PROGRAM Temp
VAR	
	H_LID				:ARRAY[1..10] OF Temp_controller;
	H_CHAMBER			:ARRAY[1..10] OF Temp_controller;
	H_PEN_VALVE			:Temp_controller;
	H_GATE_VALVE		:Temp_controller;
	H_IGS				:ARRAY[1..10] OF Temp_controller;
	H_TAPE				:ARRAY[1..10] OF Temp_controller;
	H_FORELINE			:ARRAY[1..20] OF Temp_controller;
	H_STAGE				:ARRAY[1..10] OF Temp_controller;	
END_VAR

//E01 PEN_VALVE PID		
	IF 	GV.AI.APC_Temp-GV.AO.APC_Temp_SV<3	
	THEN 
		H_PEN_VALVE.PID_Feedforward:=GV_H.PEN_VALVE_HEATER_PID.Feedforward;
	ELSE
		H_PEN_VALVE.PID_Feedforward:=0;
	END_IF	
	H_PEN_VALVE(
		ENABLE:= GV.AI.APC_Temp<110, 
		AUTO_TUNE:= GV.PEN_VALVE_HEATER_AUTO_TUNE_EN, 
		AUTO_TUNE_OUTPUT:=GV.PEN_VALVE_HEATER_AUTO_TUNE_OUTPUT,
		TEMP_SV:= GV.AO.APC_Temp_SV, 
		TEMP_ACTUAL:= GV.AI.APC_Temp, 
		TEMP_RATE:=5,
		PID_P:= GV_H.PEN_VALVE_HEATER_PID.P, 
		PID_I:= GV_H.PEN_VALVE_HEATER_PID.I, 
		PID_D:= GV_H.PEN_VALVE_HEATER_PID.D, 
		PID_Dp:= GV_H.PEN_VALVE_HEATER_PID.DP,
		PID_Output_Limit:= GV_H.PEN_VALVE_HEATER_PID.Output_Limit,
		SSR_ON=> GV.PEN_VALVE_HEATER_SSR_ON
	);		
	IF H_PEN_VALVE.PID_AUTO_TUNE_DONE
		THEN
		GV_H.PEN_VALVE_HEATER_PID.P:=H_PEN_VALVE.PID_AUTO_TUNE_P;
		GV_H.PEN_VALVE_HEATER_PID.I:=H_PEN_VALVE.PID_AUTO_TUNE_I;
		GV_H.PEN_VALVE_HEATER_PID.D:=H_PEN_VALVE.PID_AUTO_TUNE_D;
		GV.PEN_VALVE_HEATER_AUTO_TUNE_EN:=FALSE;
	END_IF
	
//E02 LID1 PID
	H_LID[1](
	ENABLE:= GV.AI.Lid_Temp<100, 
	AUTO_TUNE:= GV.LID_HEATER_AUTO_TUNE_EN[1], 
	AUTO_TUNE_OUTPUT:=GV.LID_HEATER_AUTO_TUNE_OUTPUT[1],
	TEMP_SV:= GV.AO.LID_Temp_SV, 
	TEMP_ACTUAL:= GV.AI.Lid_Temp, 
	TEMP_RATE:=5,
	PID_P:= GV_H.LID_HEATER_PID[1].P, 
	PID_I:= GV_H.LID_HEATER_PID[1].I, 
	PID_D:= GV_H.LID_HEATER_PID[1].D, 
	PID_Dp:= GV_H.LID_HEATER_PID[1].DP, 
	PID_Feedforward:= GV_H.LID_HEATER_PID[1].Feedforward,
	PID_Output_Limit:= GV_H.LID_HEATER_PID[1].Output_Limit,
	SSR_ON=> GV.LID_HEATER_SSR_ON[1],
	SSR_ON=> GV.LID_HEATER_SSR_ON[2],
	SSR_ON=> GV.LID_HEATER_SSR_ON[3],
	SSR_ON=> GV.LID_HEATER_SSR_ON[4]
	);	
	IF H_LID[1].PID_AUTO_TUNE_DONE
		THEN
		GV_H.LID_HEATER_PID[1].P:=H_LID[1].PID_AUTO_TUNE_P;
		GV_H.LID_HEATER_PID[1].I:=H_LID[1].PID_AUTO_TUNE_I;
		GV_H.LID_HEATER_PID[1].D:=H_LID[1].PID_AUTO_TUNE_D;
		GV.LID_HEATER_AUTO_TUNE_EN[1]:=FALSE;
	END_IF
//E06 CHAMBER1 PID
	H_CHAMBER[1](
	ENABLE:= GV.AI.CHAMBER_Temp1<100, 
	AUTO_TUNE:= GV.CHAMBER_HEATER_AUTO_TUNE_EN[1], 
	AUTO_TUNE_OUTPUT:=GV.CHAMBER_HEATER_AUTO_TUNE_OUTPUT[1],
	TEMP_SV:= GV.AO.Chamber_Temp1_SV, 
	TEMP_ACTUAL:= GV.AI.CHAMBER_Temp1, 
	TEMP_RATE:=5,
	PID_P:= GV_H.CHAMBER_HEATER_PID[1].P, 
	PID_I:= GV_H.CHAMBER_HEATER_PID[1].I, 
	PID_D:= GV_H.CHAMBER_HEATER_PID[1].D, 
	PID_Dp:= GV_H.CHAMBER_HEATER_PID[1].DP, 
	PID_Feedforward:= GV_H.CHAMBER_HEATER_PID[1].Feedforward,
	PID_Output_Limit:= GV_H.CHAMBER_HEATER_PID[1].Output_Limit,
	SSR_ON=> GV.CHAMBER_HEATER_SSR_ON[1]
	);	
	IF H_CHAMBER[1].PID_AUTO_TUNE_DONE
		THEN
		GV_H.CHAMBER_HEATER_PID[1].P:=H_CHAMBER[1].PID_AUTO_TUNE_P;
		GV_H.CHAMBER_HEATER_PID[1].I:=H_CHAMBER[1].PID_AUTO_TUNE_I;
		GV_H.CHAMBER_HEATER_PID[1].D:=H_CHAMBER[1].PID_AUTO_TUNE_D;
		GV.CHAMBER_HEATER_AUTO_TUNE_EN[1]:=FALSE;
	END_IF
//E07 CHAMBER2 PID	
	H_CHAMBER[2](
	ENABLE:= GV.AI.CHAMBER_Temp2<100, 
	AUTO_TUNE:= GV.CHAMBER_HEATER_AUTO_TUNE_EN[2], 
	AUTO_TUNE_OUTPUT:=GV.CHAMBER_HEATER_AUTO_TUNE_OUTPUT[2],
	TEMP_SV:= GV.AO.Chamber_Temp2_SV, 
	TEMP_ACTUAL:= GV.AI.CHAMBER_Temp2, 
	TEMP_RATE:=5,
	PID_P:= GV_H.CHAMBER_HEATER_PID[2].P, 
	PID_I:= GV_H.CHAMBER_HEATER_PID[2].I, 
	PID_D:= GV_H.CHAMBER_HEATER_PID[2].D, 
	PID_Dp:= GV_H.CHAMBER_HEATER_PID[2].DP, 
	PID_Feedforward:= GV_H.CHAMBER_HEATER_PID[2].Feedforward,
	PID_Output_Limit:= GV_H.CHAMBER_HEATER_PID[2].Output_Limit,
	SSR_ON=> GV.CHAMBER_HEATER_SSR_ON[2]
	);	
	IF H_CHAMBER[2].PID_AUTO_TUNE_DONE
		THEN
		GV_H.CHAMBER_HEATER_PID[2].P:=H_CHAMBER[2].PID_AUTO_TUNE_P;
		GV_H.CHAMBER_HEATER_PID[2].I:=H_CHAMBER[2].PID_AUTO_TUNE_I;
		GV_H.CHAMBER_HEATER_PID[2].D:=H_CHAMBER[2].PID_AUTO_TUNE_D;
		GV.CHAMBER_HEATER_AUTO_TUNE_EN[2]:=FALSE;
	END_IF
(*
	//E08 CHAMBER3 PID		
	H_CHAMBER[3](
	ENABLE:= GV.AI.CHAMBER_Temp3<100, 
	AUTO_TUNE:= GV.CHAMBER_HEATER_AUTO_TUNE_EN[3], 
	AUTO_TUNE_OUTPUT:=GV.CHAMBER_HEATER_AUTO_TUNE_OUTPUT[3],
	TEMP_SV:= GV.AO.Chamber_Temp3_SV, 
	TEMP_ACTUAL:= GV.AI.Chamber_Temp3, 
	PID_P:= GV_H.CHAMBER_HEATER_PID[3].P, 
	PID_I:= GV_H.CHAMBER_HEATER_PID[3].I, 
	PID_D:= GV_H.CHAMBER_HEATER_PID[3].D, 
	PID_Dp:= GV_H.CHAMBER_HEATER_PID[3].DP,
	PID_Feedforward:= GV_H.CHAMBER_HEATER_PID[3].Feedforward,
	PID_Output_Limit:= GV_H.CHAMBER_HEATER_PID[3].Output_Limit,
	SSR_ON=> GV.CHAMBER_HEATER_SSR_ON[4]
	);	
	IF H_CHAMBER[3].PID_AUTO_TUNE_DONE
		THEN
		GV_H.CHAMBER_HEATER_PID[3].P:=H_CHAMBER[3].PID_AUTO_TUNE_P;
		GV_H.CHAMBER_HEATER_PID[3].I:=H_CHAMBER[3].PID_AUTO_TUNE_I;
		GV_H.CHAMBER_HEATER_PID[3].D:=H_CHAMBER[3].PID_AUTO_TUNE_D;
		GV.CHAMBER_HEATER_AUTO_TUNE_EN[3]:=FALSE;
	END_IF

	//E18 GATE VALVE PID
		IF 	ABS(GV.AI.GATE_VALVE_Temp-GV.AO.Gate_Valve_Temp_SV)<5	
		THEN 
			H_GATE_VALVE.PID_Feedforward:=GV_H.GATE_VALVE_HEATER_PID.Feedforward;
		ELSE
			H_GATE_VALVE.PID_Feedforward:=0;
		END_IF
		H_GATE_VALVE(
		ENABLE:= GV.AI.GATE_VALVE_Temp<100, 
		AUTO_TUNE:= GV.GATE_VALVE_HEATER_AUTO_TUNE_EN, 
		AUTO_TUNE_OUTPUT:=GV.GATE_VALVE_HEATER_AUTO_TUNE_OUTPUT,
		TEMP_SV:= GV.AO.Gate_Valve_Temp_SV, 
		TEMP_ACTUAL:= GV.AI.GATE_VALVE_Temp, 
		PID_P:= GV_H.GATE_VALVE_HEATER_PID.P, 
		PID_I:= GV_H.GATE_VALVE_HEATER_PID.I, 
		PID_D:= GV_H.GATE_VALVE_HEATER_PID.D, 
		PID_Dp:= GV_H.GATE_VALVE_HEATER_PID.DP, 
		PID_Output_Limit:= GV_H.GATE_VALVE_HEATER_PID.Output_Limit,
		SSR_ON=> GV.GATE_VALVE_SSR_ON
		);		
		IF H_GATE_VALVE.PID_AUTO_TUNE_DONE
			THEN
			GV_H.GATE_VALVE_HEATER_PID.P:=H_GATE_VALVE.PID_AUTO_TUNE_P;
			GV_H.GATE_VALVE_HEATER_PID.I:=H_GATE_VALVE.PID_AUTO_TUNE_I;
			GV_H.GATE_VALVE_HEATER_PID.D:=H_GATE_VALVE.PID_AUTO_TUNE_D;
			GV.GATE_VALVE_HEATER_AUTO_TUNE_EN:=FALSE;
		END_IF	
		
	//E31	TAPE1 PID		
		H_TAPE[1](
		ENABLE:= GV.AI.TAPE_Temp1<120, 
		AUTO_TUNE:= GV.TAPE_HEATER_AUTO_TUNE_EN[1],
		AUTO_TUNE_OUTPUT:=GV.TAPE_HEATER_AUTO_TUNE_OUTPUT[1], 
		TEMP_SV:= GV.AO.Tape_Temp1_SV, 
		TEMP_ACTUAL:= GV.AI.TAPE_Temp1, 
		PID_P:= GV_H.TAPE_HEATER_PID[1].P, 
		PID_I:= GV_H.TAPE_HEATER_PID[1].I, 
		PID_D:= GV_H.TAPE_HEATER_PID[1].D, 
		PID_Dp:= GV_H.TAPE_HEATER_PID[1].DP, 
		PID_Feedforward:= ,
		PID_Output_Limit:= GV_H.TAPE_HEATER_PID[1].Output_Limit,
		SSR_ON=> GV.TAPE_HEATER_SSR_ON[1]
		);	
		IF H_TAPE[1].PID_AUTO_TUNE_DONE
			THEN
			GV_H.TAPE_HEATER_PID[1].P:=H_TAPE[1].PID_AUTO_TUNE_P;
			GV_H.TAPE_HEATER_PID[1].I:=H_TAPE[1].PID_AUTO_TUNE_I;
			GV_H.TAPE_HEATER_PID[1].D:=H_TAPE[1].PID_AUTO_TUNE_D;
			GV.TAPE_HEATER_AUTO_TUNE_EN[1]:=FALSE;
		END_IF
	//E32	TAPE2 PID		
		H_TAPE[2](
		ENABLE:= GV.AI.TAPE_Temp2<120, 
		AUTO_TUNE:= GV.TAPE_HEATER_AUTO_TUNE_EN[2], 
		AUTO_TUNE_OUTPUT:=GV.TAPE_HEATER_AUTO_TUNE_OUTPUT[2], 
		TEMP_SV:= GV.AO.Tape_Temp2_SV, 
		TEMP_ACTUAL:= GV.AI.TAPE_Temp2, 
		PID_P:= GV_H.TAPE_HEATER_PID[2].P, 
		PID_I:= GV_H.TAPE_HEATER_PID[2].I, 
		PID_D:= GV_H.TAPE_HEATER_PID[2].D, 
		PID_Dp:= GV_H.TAPE_HEATER_PID[2].DP, 
		PID_Feedforward:= ,
		PID_Output_Limit:= GV_H.TAPE_HEATER_PID[2].Output_Limit,
		SSR_ON=> GV.TAPE_HEATER_SSR_ON[2]
		);	
		IF H_TAPE[2].PID_AUTO_TUNE_DONE
			THEN
			GV_H.TAPE_HEATER_PID[2].P:=H_TAPE[2].PID_AUTO_TUNE_P;
			GV_H.TAPE_HEATER_PID[2].I:=H_TAPE[2].PID_AUTO_TUNE_I;
			GV_H.TAPE_HEATER_PID[2].D:=H_TAPE[2].PID_AUTO_TUNE_D;
			GV.TAPE_HEATER_AUTO_TUNE_EN[2]:=FALSE;
		END_IF
	//E35	IGS1 PID		
		H_IGS[1](
		ENABLE:= GV.AI.IGS_Temp1<50, 
		AUTO_TUNE:= GV.IGS_HEATER_AUTO_TUNE_EN[1], 
		AUTO_TUNE_OUTPUT:=GV.IGS_HEATER_AUTO_TUNE_OUTPUT[1], 
		TEMP_SV:= GV.AO.IGS_Temp1_SV, 
		TEMP_ACTUAL:= GV.AI.IGS_Temp1, 
		PID_P:= GV_H.IGS_HEATER_PID[1].P, 
		PID_I:= GV_H.IGS_HEATER_PID[1].I, 
		PID_D:= GV_H.IGS_HEATER_PID[1].D, 
		PID_Dp:= GV_H.IGS_HEATER_PID[1].DP, 
		PID_Feedforward:= GV_H.IGS_HEATER_PID[1].Feedforward,
		PID_Output_Limit:= GV_H.IGS_HEATER_PID[1].Output_Limit,
		SSR_ON=> GV.IGS_HEATER_SSR_ON[1]
		);	
		IF H_IGS[1].PID_AUTO_TUNE_DONE
			THEN
			GV_H.IGS_HEATER_PID[1].P:=H_IGS[1].PID_AUTO_TUNE_P;
			GV_H.IGS_HEATER_PID[1].I:=H_IGS[1].PID_AUTO_TUNE_I;
			GV_H.IGS_HEATER_PID[1].D:=H_IGS[1].PID_AUTO_TUNE_D;
			GV.IGS_HEATER_AUTO_TUNE_EN[1]:=FALSE;
		END_IF
	//E36	IGS2 PID	
		IF 	GV.AI.IGS_Temp2>GV.AO.IGS_Temp2_SV+3 THEN 
			H_IGS[2].PID_Feedforward:=0;
			ELSE
				H_IGS[2].PID_Feedforward:=GV_H.IGS_HEATER_PID[2].Feedforward;
		
		END_IF
		H_IGS[2](
		ENABLE:= GV.AI.IGS_Temp2<50, 
		AUTO_TUNE:= GV.IGS_HEATER_AUTO_TUNE_EN[2], 
		AUTO_TUNE_OUTPUT:=GV.IGS_HEATER_AUTO_TUNE_OUTPUT[2],
		TEMP_SV:= GV.AO.IGS_Temp2_SV, 
		TEMP_ACTUAL:= GV.AI.IGS_Temp2, 
		TEMP_RATE:=10,
		PID_P:= GV_H.IGS_HEATER_PID[2].P, 
		PID_I:= GV_H.IGS_HEATER_PID[2].I, 
		PID_D:= GV_H.IGS_HEATER_PID[2].D, 
		PID_Dp:= GV_H.IGS_HEATER_PID[2].DP, 
		PID_Feedforward:= ,
		PID_Output_Limit:= GV_H.IGS_HEATER_PID[2].Output_Limit,
		SSR_ON=> GV.IGS_HEATER_SSR_ON[2]
		);	
		IF H_IGS[2].PID_AUTO_TUNE_DONE
			THEN
			GV_H.IGS_HEATER_PID[2].P:=H_IGS[2].PID_AUTO_TUNE_P;
			GV_H.IGS_HEATER_PID[2].I:=H_IGS[2].PID_AUTO_TUNE_I;
			GV_H.IGS_HEATER_PID[2].D:=H_IGS[2].PID_AUTO_TUNE_D;
			GV.IGS_HEATER_AUTO_TUNE_EN[2]:=FALSE;
		END_IF
*)	
//FORELINE1 PID	SSR7	AV105	
	H_FORELINE[1](
	ENABLE:= GV.AI.AV105_Temp<120, 
	AUTO_TUNE:= GV.FORELINE_HEATER_AUTO_TUNE_EN[1], 
	AUTO_TUNE_OUTPUT:=GV.FORELINE_HEATER_AUTO_TUNE_OUTPUT[1],
	TEMP_SV:= GV.AO.AV105_Temp_SV, 
	TEMP_ACTUAL:= GV.AI.AV105_Temp, 
	TEMP_RATE:=10,
	PID_P:= GV_H.FORELINE_HEATER_PID[1].P, 
	PID_I:= GV_H.FORELINE_HEATER_PID[1].I, 
	PID_D:= GV_H.FORELINE_HEATER_PID[1].D, 
	PID_Dp:= GV_H.FORELINE_HEATER_PID[1].DP, 
	PID_Feedforward:= GV_H.FORELINE_HEATER_PID[1].Feedforward,
	PID_Output_Limit:= GV_H.FORELINE_HEATER_PID[1].Output_Limit,
	SSR_ON=> GV.FORELINE_HEATER_SSR_ON[1]);
	
	IF H_FORELINE[1].PID_AUTO_TUNE_DONE
		THEN
		GV_H.FORELINE_HEATER_PID[1].P:=H_FORELINE[1].PID_AUTO_TUNE_P;
		GV_H.FORELINE_HEATER_PID[1].I:=H_FORELINE[1].PID_AUTO_TUNE_I;
		GV_H.FORELINE_HEATER_PID[1].D:=H_FORELINE[1].PID_AUTO_TUNE_D;
		GV.FORELINE_HEATER_AUTO_TUNE_EN[1]:=FALSE;
	END_IF
//FORELINE2 PID		SSR8	AV104
	H_FORELINE[2](
	ENABLE:= GV.AI.AV104_Temp<120, 
	AUTO_TUNE:= GV.FORELINE_HEATER_AUTO_TUNE_EN[2], 
	AUTO_TUNE_OUTPUT:=GV.FORELINE_HEATER_AUTO_TUNE_OUTPUT[2],
	TEMP_SV:= GV.AO.AV104_Temp_SV, 
	TEMP_ACTUAL:= GV.AI.AV104_Temp,
	TEMP_RATE:=10, 
	PID_P:= GV_H.FORELINE_HEATER_PID[2].P, 
	PID_I:= GV_H.FORELINE_HEATER_PID[2].I, 
	PID_D:= GV_H.FORELINE_HEATER_PID[2].D, 
	PID_Dp:= GV_H.FORELINE_HEATER_PID[2].DP, 
	PID_Feedforward:= GV_H.FORELINE_HEATER_PID[2].Feedforward,
	PID_Output_Limit:= GV_H.FORELINE_HEATER_PID[2].Output_Limit,
	SSR_ON=> GV.FORELINE_HEATER_SSR_ON[2]);
	
	IF H_FORELINE[2].PID_AUTO_TUNE_DONE
		THEN
		GV_H.FORELINE_HEATER_PID[2].P:=H_FORELINE[2].PID_AUTO_TUNE_P;
		GV_H.FORELINE_HEATER_PID[2].I:=H_FORELINE[2].PID_AUTO_TUNE_I;
		GV_H.FORELINE_HEATER_PID[2].D:=H_FORELINE[2].PID_AUTO_TUNE_D;
		GV.FORELINE_HEATER_AUTO_TUNE_EN[2]:=FALSE;
	END_IF
//FORELINE3 PID		SSR9	AV102
IF GV.AI.AV102_Temp<GV.AO.AV102_Temp_SV+1
	THEN 
	GV_H.FORELINE_HEATER_PID[3].Feedforward:=8.5;
	ELSE
	GV_H.FORELINE_HEATER_PID[3].Feedforward:=0;
END_IF
	H_FORELINE[3](
	ENABLE:= GV.AI.AV102_Temp<120, 
	AUTO_TUNE:= GV.FORELINE_HEATER_AUTO_TUNE_EN[3], 
	AUTO_TUNE_OUTPUT:=GV.FORELINE_HEATER_AUTO_TUNE_OUTPUT[3],
	TEMP_SV:= GV.AO.AV102_Temp_SV, 
	TEMP_ACTUAL:= GV.AI.AV102_Temp,
	TEMP_RATE:=10, 
	PID_P:= GV_H.FORELINE_HEATER_PID[3].P, 
	PID_I:= GV_H.FORELINE_HEATER_PID[3].I, 
	PID_D:= GV_H.FORELINE_HEATER_PID[3].D, 
	PID_Dp:= GV_H.FORELINE_HEATER_PID[3].DP, 
	PID_Feedforward:= GV_H.FORELINE_HEATER_PID[3].Feedforward,
	PID_Output_Limit:= GV_H.FORELINE_HEATER_PID[3].Output_Limit,
	SSR_ON=> GV.FORELINE_HEATER_SSR_ON[3]);
	
	IF H_FORELINE[3].PID_AUTO_TUNE_DONE
		THEN
		GV_H.FORELINE_HEATER_PID[3].P:=H_FORELINE[3].PID_AUTO_TUNE_P;
		GV_H.FORELINE_HEATER_PID[3].I:=H_FORELINE[3].PID_AUTO_TUNE_I;
		GV_H.FORELINE_HEATER_PID[3].D:=H_FORELINE[3].PID_AUTO_TUNE_D;
		GV.FORELINE_HEATER_AUTO_TUNE_EN[3]:=FALSE;
	END_IF	
//FORELINE4 PID		SSR10	AV101
	H_FORELINE[4](
	ENABLE:= GV.AI.AV101_Temp<120, 
	AUTO_TUNE:= GV.FORELINE_HEATER_AUTO_TUNE_EN[4],
	AUTO_TUNE_OUTPUT:=GV.FORELINE_HEATER_AUTO_TUNE_OUTPUT[4], 
	TEMP_SV:= GV.AO.AV101_Temp_SV, 
	TEMP_ACTUAL:= GV.AI.AV101_Temp, 
	TEMP_RATE:=10,
	PID_P:= GV_H.FORELINE_HEATER_PID[4].P, 
	PID_I:= GV_H.FORELINE_HEATER_PID[4].I, 
	PID_D:= GV_H.FORELINE_HEATER_PID[4].D, 
	PID_Dp:= GV_H.FORELINE_HEATER_PID[4].DP, 
	PID_Feedforward:= GV_H.FORELINE_HEATER_PID[4].Feedforward,
	PID_Output_Limit:= GV_H.FORELINE_HEATER_PID[4].Output_Limit,
	SSR_ON=> GV.FORELINE_HEATER_SSR_ON[4]);
	
	IF H_FORELINE[4].PID_AUTO_TUNE_DONE
		THEN
		GV_H.FORELINE_HEATER_PID[4].P:=H_FORELINE[4].PID_AUTO_TUNE_P;
		GV_H.FORELINE_HEATER_PID[4].I:=H_FORELINE[4].PID_AUTO_TUNE_I;
		GV_H.FORELINE_HEATER_PID[4].D:=H_FORELINE[4].PID_AUTO_TUNE_D;
		GV.FORELINE_HEATER_AUTO_TUNE_EN[4]:=FALSE;
	END_IF
//FORELINE5 PID		SS11	Exh1-3
	H_FORELINE[5](
	ENABLE:= GV.AI.Exhaust1_3_Temp<120, 
	AUTO_TUNE:= GV.FORELINE_HEATER_AUTO_TUNE_EN[5], 
	AUTO_TUNE_OUTPUT:=GV.FORELINE_HEATER_AUTO_TUNE_OUTPUT[5],
	TEMP_SV:= GV.AO.Exhaust1_3_Temp_SV ,
	TEMP_ACTUAL:= GV.AI.Exhaust1_3_Temp,
	TEMP_RATE:=10, 
	PID_P:= GV_H.FORELINE_HEATER_PID[5].P, 
	PID_I:= GV_H.FORELINE_HEATER_PID[5].I, 
	PID_D:= GV_H.FORELINE_HEATER_PID[5].D, 
	PID_Dp:= GV_H.FORELINE_HEATER_PID[5].DP, 
	PID_Feedforward:= GV_H.FORELINE_HEATER_PID[5].Feedforward,
	PID_Output_Limit:= GV_H.FORELINE_HEATER_PID[5].Output_Limit,
	SSR_ON=> GV.FORELINE_HEATER_SSR_ON[5]);
	
	IF H_FORELINE[5].PID_AUTO_TUNE_DONE
		THEN
		GV_H.FORELINE_HEATER_PID[5].P:=H_FORELINE[5].PID_AUTO_TUNE_P;
		GV_H.FORELINE_HEATER_PID[5].I:=H_FORELINE[5].PID_AUTO_TUNE_I;
		GV_H.FORELINE_HEATER_PID[5].D:=H_FORELINE[5].PID_AUTO_TUNE_D;
		GV.FORELINE_HEATER_AUTO_TUNE_EN[5]:=FALSE;
	END_IF
//FORELINE6 PID		SS12	Exh4-7
	H_FORELINE[6](
	ENABLE:= GV.AI.Exhaust4_7_Temp<120, 
	AUTO_TUNE:= GV.FORELINE_HEATER_AUTO_TUNE_EN[6], 
	TEMP_SV:= GV.AO.Exhaust4_7_Temp_SV, 
	TEMP_ACTUAL:= GV.AI.Exhaust4_7_Temp,
	TEMP_RATE:=10, 
	PID_P:= GV_H.FORELINE_HEATER_PID[6].P, 
	PID_I:= GV_H.FORELINE_HEATER_PID[6].I, 
	PID_D:= GV_H.FORELINE_HEATER_PID[6].D, 
	PID_Dp:= GV_H.FORELINE_HEATER_PID[6].DP, 
	PID_Feedforward:= GV_H.FORELINE_HEATER_PID[6].Feedforward,
	PID_Output_Limit:= GV_H.FORELINE_HEATER_PID[6].Output_Limit,
	SSR_ON=> GV.FORELINE_HEATER_SSR_ON[6]);
	
	IF H_FORELINE[6].PID_AUTO_TUNE_DONE
		THEN
		GV_H.FORELINE_HEATER_PID[6].P:=H_FORELINE[6].PID_AUTO_TUNE_P;
		GV_H.FORELINE_HEATER_PID[6].I:=H_FORELINE[6].PID_AUTO_TUNE_I;
		GV_H.FORELINE_HEATER_PID[6].D:=H_FORELINE[6].PID_AUTO_TUNE_D;
		GV.FORELINE_HEATER_AUTO_TUNE_EN[6]:=FALSE;
	END_IF	
//H-STAGE1
IF (GV.AI.Stage_Temp1-GV.AO.Stage_Temp1_SV)<3 AND GV.AO.Stage_Temp1_SV>100
	THEN
	GV_H.STAGE_HEATER_PID[1].Feedforward:=9.5;
	ELSE
		GV_H.STAGE_HEATER_PID[1].Feedforward:=0;
END_IF
	H_STAGE[1](
	ENABLE:= GV.AI.Stage_Temp1<250 AND PM.NDI.Lid_Closed, 
	AUTO_TUNE:= GV.STAGE_HEATER_AUTO_TUNE_EN[1], 
	TEMP_SV:= GV.AO.Stage_Temp1_SV, 
	TEMP_ACTUAL:= GV.AI.Stage_Temp1,
	TEMP_RATE:=10, 
	PID_P:= GV_H.STAGE_HEATER_PID[1].P, 
	PID_I:= GV_H.STAGE_HEATER_PID[1].I, 
	PID_D:= GV_H.STAGE_HEATER_PID[1].D, 
	PID_Dp:= GV_H.STAGE_HEATER_PID[1].DP, 
	PID_Feedforward:= GV_H.STAGE_HEATER_PID[1].Feedforward,
	PID_Output_Limit:= GV_H.STAGE_HEATER_PID[1].Output_Limit,
	SCR_OUT=> GV.STAGE_HEATER_SCR_OUTPUT[1]);
		
	IF H_STAGE[1].TEMP_ACTUAL>=H_STAGE[1].TEMP_SV	THEN GV.STAGE_HEATER_SCR_OUTPUT[1]:=H_STAGE[1].PID_Feedforward;END_IF;
	
	IF H_STAGE[1].PID_AUTO_TUNE_DONE
		THEN
		GV_H.STAGE_HEATER_PID[1].P:=H_STAGE[1].PID_AUTO_TUNE_P;
		GV_H.STAGE_HEATER_PID[1].I:=H_STAGE[1].PID_AUTO_TUNE_I;
		GV_H.STAGE_HEATER_PID[1].D:=H_STAGE[1].PID_AUTO_TUNE_D;
		GV.STAGE_HEATER_AUTO_TUNE_EN[1]:=FALSE;
	END_IF
	
//H-STAGE2
	H_STAGE[2](
	ENABLE:= GV.AI.Stage_Temp2<250 AND PM.NDI.Lid_Closed, 
	AUTO_TUNE:= GV.STAGE_HEATER_AUTO_TUNE_EN[2], 
	TEMP_SV:= GV.AO.Stage_Temp2_SV, 
	TEMP_ACTUAL:= GV.AI.Stage_Temp2, 
	TEMP_RATE:=10,
	PID_P:= GV_H.STAGE_HEATER_PID[2].P, 
	PID_I:= GV_H.STAGE_HEATER_PID[2].I, 
	PID_D:= GV_H.STAGE_HEATER_PID[2].D, 
	PID_Dp:= GV_H.STAGE_HEATER_PID[2].DP, 
	PID_Feedforward:= GV_H.STAGE_HEATER_PID[2].Feedforward,
	PID_Output_Limit:= GV_H.STAGE_HEATER_PID[2].Output_Limit,
	SCR_OUT=> GV.STAGE_HEATER_SCR_OUTPUT[2]);

	IF H_STAGE[2].TEMP_ACTUAL>=H_STAGE[2].TEMP_SV	THEN GV.STAGE_HEATER_SCR_OUTPUT[2]:=H_STAGE[2].PID_Feedforward;END_IF;
	
	IF H_STAGE[2].PID_AUTO_TUNE_DONE
		THEN
		GV_H.STAGE_HEATER_PID[2].P:=H_STAGE[2].PID_AUTO_TUNE_P;
		GV_H.STAGE_HEATER_PID[2].I:=H_STAGE[2].PID_AUTO_TUNE_I;
		GV_H.STAGE_HEATER_PID[2].D:=H_STAGE[2].PID_AUTO_TUNE_D;
		GV.STAGE_HEATER_AUTO_TUNE_EN[2]:=FALSE;
	END_IF
	
//H-STAGE3
IF (GV.AI.Stage_Temp3-GV.AO.Stage_Temp3_SV)<3 AND GV.AO.Stage_Temp3_SV>100
	THEN
	GV_H.STAGE_HEATER_PID[3].Feedforward:=8;
	ELSE
		GV_H.STAGE_HEATER_PID[3].Feedforward:=0;
END_IF
	H_STAGE[3](
	ENABLE:= GV.AI.Stage_Temp3<250 AND PM.NDI.Lid_Closed, 
	AUTO_TUNE:= GV.STAGE_HEATER_AUTO_TUNE_EN[3], 
	TEMP_SV:= GV.AO.Stage_Temp3_SV, 
	TEMP_ACTUAL:= GV.AI.Stage_Temp3, 
	TEMP_RATE:=10,
	PID_P:= GV_H.STAGE_HEATER_PID[3].P, 
	PID_I:= GV_H.STAGE_HEATER_PID[3].I, 
	PID_D:= GV_H.STAGE_HEATER_PID[3].D, 
	PID_Dp:= GV_H.STAGE_HEATER_PID[3].DP, 
	PID_Feedforward:= GV_H.STAGE_HEATER_PID[3].Feedforward,
	PID_Output_Limit:= GV_H.STAGE_HEATER_PID[3].Output_Limit,
	SCR_OUT=> GV.STAGE_HEATER_SCR_OUTPUT[3]);

	IF H_STAGE[3].TEMP_ACTUAL>=H_STAGE[3].TEMP_SV	THEN GV.STAGE_HEATER_SCR_OUTPUT[3]:=H_STAGE[3].PID_Feedforward;END_IF;
	
	IF H_STAGE[3].PID_AUTO_TUNE_DONE
		THEN
		GV_H.STAGE_HEATER_PID[3].P:=H_STAGE[3].PID_AUTO_TUNE_P;
		GV_H.STAGE_HEATER_PID[3].I:=H_STAGE[3].PID_AUTO_TUNE_I;
		GV_H.STAGE_HEATER_PID[3].D:=H_STAGE[3].PID_AUTO_TUNE_D;
		GV.STAGE_HEATER_AUTO_TUNE_EN[3]:=FALSE;
	END_IF
	
//H-STAGE4
	H_STAGE[4](
	ENABLE:= GV.AI.Stage_Temp4<250 AND PM.NDI.Lid_Closed, 
	AUTO_TUNE:= GV.STAGE_HEATER_AUTO_TUNE_EN[4], 
	TEMP_SV:= GV.AO.Stage_Temp4_SV, 
	TEMP_ACTUAL:= GV.AI.Stage_Temp4, 
	TEMP_RATE:=10,
	PID_P:= GV_H.STAGE_HEATER_PID[4].P, 
	PID_I:= GV_H.STAGE_HEATER_PID[4].I, 
	PID_D:= GV_H.STAGE_HEATER_PID[4].D, 
	PID_Dp:= GV_H.STAGE_HEATER_PID[4].DP, 
	PID_Feedforward:= GV_H.STAGE_HEATER_PID[4].Feedforward,
	PID_Output_Limit:= GV_H.STAGE_HEATER_PID[4].Output_Limit,
	SCR_OUT=> GV.STAGE_HEATER_SCR_OUTPUT[4]);

	IF H_STAGE[4].TEMP_ACTUAL>=H_STAGE[4].TEMP_SV	THEN GV.STAGE_HEATER_SCR_OUTPUT[4]:=H_STAGE[4].PID_Feedforward;END_IF;
	
	IF H_STAGE[4].PID_AUTO_TUNE_DONE
		THEN
		GV_H.STAGE_HEATER_PID[4].P:=H_STAGE[4].PID_AUTO_TUNE_P;
		GV_H.STAGE_HEATER_PID[4].I:=H_STAGE[4].PID_AUTO_TUNE_I;
		GV_H.STAGE_HEATER_PID[4].D:=H_STAGE[4].PID_AUTO_TUNE_D;
		GV.STAGE_HEATER_AUTO_TUNE_EN[4]:=FALSE;
	END_IF

END_PROGRAM
